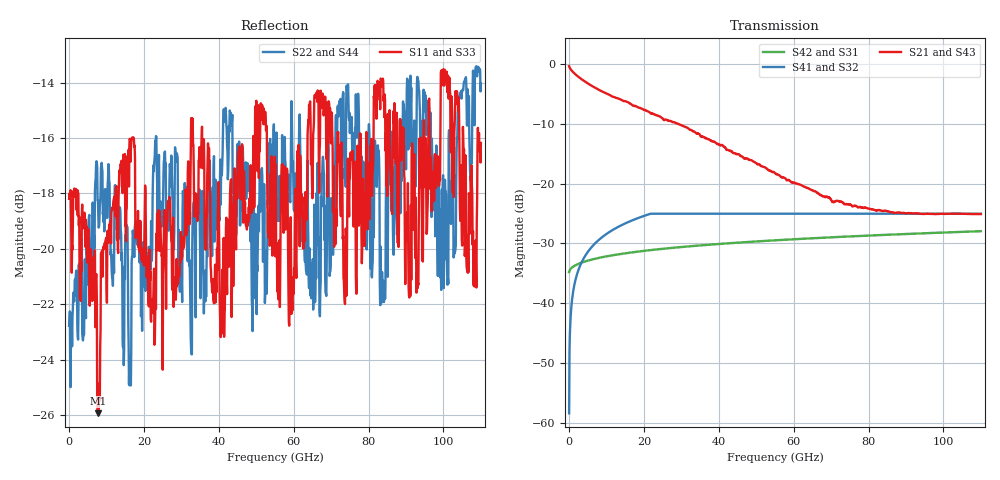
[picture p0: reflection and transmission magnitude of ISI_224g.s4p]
! Created with skrf 1.10.0 (http://scikit-rf.org).
# GHz S RI R 50.0
!freq ReS11 ImS11 ReS12 ImS12 ReS13 ImS13
! ReS14 ImS14
! ReS21 ImS21 ReS22 ImS22 ReS23 ImS23
! ReS24 ImS24
! ReS31 ImS31 ReS32 ImS32 ReS33 ImS33
! ReS34 ImS34
! ReS41 ImS41 ReS42 ImS42 ReS43 ImS43
! ReS44 ImS44
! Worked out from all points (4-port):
!   1101 points, 10 MHz to 110 GHz, reference 50 ohm
!   strongest paths, dB at 10 MHz, 27.51 GHz, 55.01 GHz, 82.5 GHz, 110 GHz:
!     S21: -0.4, -9.7, -18.3, -24.4, -25.1
!     S43: -0.4, -9.7, -18.3, -24.4, -25.0
!     S41: -58.4, -25.0, -25.0, -25.0, -25.0
!     S32: -58.4, -25.0, -25.0, -25.0, -25.0
!     S42: -34.8, -30.8, -29.5, -28.6, -28.0
!     S31: -34.8, -30.8, -29.5, -28.6, -28.0
!   lowest |S11| = -25.9 dB at 7.709 GHz (marker M1), VSWR 1.11, Z = 48.2 + j4.6 ohm
!   |S11| at or under -10 dB: start of sweep to end of sweep
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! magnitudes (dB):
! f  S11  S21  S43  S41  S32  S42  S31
! 10 MHz  -18.2  -0.4  -0.4  -58.4  -58.4  -34.8  -34.8
! 1.61 GHz  -18.0  -1.7  -1.7  -36.3  -36.3  -33.7  -33.7
! 7.709 GHz  -25.9  -4.2  -4.2  -29.5  -29.5  -32.5  -32.5
! 17.01 GHz  -16.0  -6.9  -7.0  -26.1  -26.1  -31.5  -31.5
! 40.71 GHz  -23.1  -13.5  -13.6  -25.0  -25.0  -30.1  -30.1
! 83.8 GHz  -13.9  -24.6  -24.5  -25.0  -25.0  -28.6  -28.6
! 110 GHz  -16.2  -25.1  -25.0  -25.0  -25.0  -28.0  -28.0
